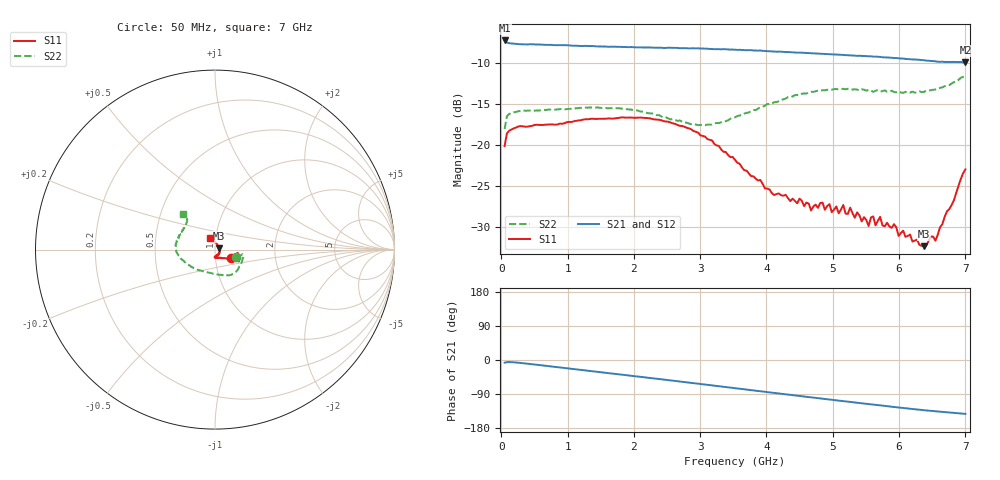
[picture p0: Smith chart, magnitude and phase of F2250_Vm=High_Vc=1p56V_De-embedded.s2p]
! Integrated Device Technology
! Corporate Headquarters
! 6024 Silver Creek Valley Road
! San Jose, CA 95138  USA
! Phone:  1-408-284-8200
! Toll Free:  1-800-223-1366
! Webpage:  http://www.idt.com/
! Timing and RF Division
! 515 Groton Road, Suite 102
! Westford, MA 01886-6024
! Device:  F2250
! Description: Voltage Variable RF Attenuator
! Frequency:  50.0 -  6000.00 MHz
! Package:  3x3 mm Thin QFN Plastic Package: 16 pin
! Ports:  2 RF, 3 DC
!  Pin  1  = GND
!  Pin  2  = NC
!  Pin  3  = RF1  = Port 1
!  Pin  4  = NC
!  Pin  5  = GND
!  Pin  6  = GND
!  Pin  7  = GND
!  Pin  8  = GND
!  Pin  9  = NC
!  Pin 10  = RF2  = Port 2
!  Pin 11  = NC
!  Pin 12  = GND
!  Pin 13  = GND
!  Pin 14  = VCNTRL
!  Pin 15  = VDD
!  Pin 16  = VMODE
! Vcntrl:  1.560 Volts
! Vmode:  +3.300 Volts
! Vdd:  +3.30  Volts
! Current:  1.330 mA
! Data:  The device was measured on a the F2250 evaluation board which has
!  individual transmission lines to the RF pins.  Data was collected
!  using a calibrated network analyzer.  The evaluation board was
!  de-embedded using a TRL calibration technique.
!  The reference plane is the edge of the package pin.
! Misc:  SN 10
!  Action Tracker AT0258
! Date Measured:  2014-11-26
! Date:  2015-10-15  MJV
! Note:
!  Integrated Device Technology supplies this data as a sample of measured
!  data at the package pin for this product.  Your particular data for this
!  product may vary.
!  Data was taken at 25 degrees C.
!  Integrated Device Technology reserves the right to change this data at anytime.
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# GHz S dB R 50
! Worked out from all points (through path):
!   201 points, 50 MHz to 7 GHz, reference 50 ohm
!   highest |S21| = -7.19 dB at 50 MHz (marker M1); lowest = -9.9 dB at 7 GHz (marker M2)
!   group delay of S21, straight-line fit = 56.9 ps
!   lowest |S11| = -32.4 dB at 6.375 GHz (marker M3), VSWR 1.05, Z = 52.3 + j0.765 ohm
!   |S11| at or under -10 dB: start of sweep to end of sweep
!   |S22| runs from -18.0 to -11.5 dB; largest |S21 - S12| = 0.0024
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0.05  -20.12 -28.5  -7.19 -7.2  -7.22 -7.2  -18.02 -20.1
0.08475  -18.56 -14.2  -7.44 -5.6  -7.44 -5.6  -16.46 -11.3
0.2585  -17.72 -9.2  -7.64 -7.2  -7.61 -7.2  -15.87 -12.5
1.2315  -16.88 -23.3  -7.87 -26.9  -7.85 -26.9  -15.39 -42.5
2.37825  -16.89 -26.0  -8.07 -50.2  -8.09 -50.2  -16.33 -70.9
2.969  -18.48 -27.0  -8.15 -62.6  -8.17 -62.6  -17.56 -97.8
3.525  -21.80 -37.2  -8.33 -74.4  -8.32 -74.5  -16.60 -131.0
4.11575  -26.11 -65.0  -8.54 -86.9  -8.53 -87.0  -14.74 -157.7
4.7065  -27.51 -90.3  -8.76 -99.2  -8.75 -99.3  -13.48 -174.8
4.94975  -27.22 -87.2  -8.87 -104.3  -8.86 -104.3  -13.22 179.3
5.08875  -28.34 -86.4  -8.93 -107.1  -8.93 -107.2  -13.18 175.9
5.15825  -27.33 -85.7  -8.96 -108.5  -8.96 -108.6  -13.11 174.5
5.193  -28.38 -81.2  -8.99 -109.2  -8.99 -109.2  -13.17 173.5
5.2625  -27.64 -82.0  -9.02 -110.6  -9.01 -110.7  -13.12 172.2
5.5405  -29.89 -72.9  -9.12 -116.3  -9.13 -116.4  -13.25 164.5
5.61  -28.72 -63.7  -9.16 -117.6  -9.17 -117.7  -13.48 163.2
5.64475  -29.81 -64.5  -9.16 -118.4  -9.19 -118.5  -13.35 161.3
5.71425  -28.78 -60.0  -9.20 -119.8  -9.24 -119.8  -13.46 160.4
5.85325  -29.93 -50.0  -9.28 -122.5  -9.29 -122.6  -13.45 155.9
6.3745  -32.36 17.6  -9.61 -132.6  -9.60 -132.6  -13.49 139.6
6.54825  -31.69 55.6  -9.74 -135.4  -9.76 -135.5  -13.19 135.5
7  -22.96 114.8  -9.86 -142.2  -9.86 -142.3  -11.47 131.4
